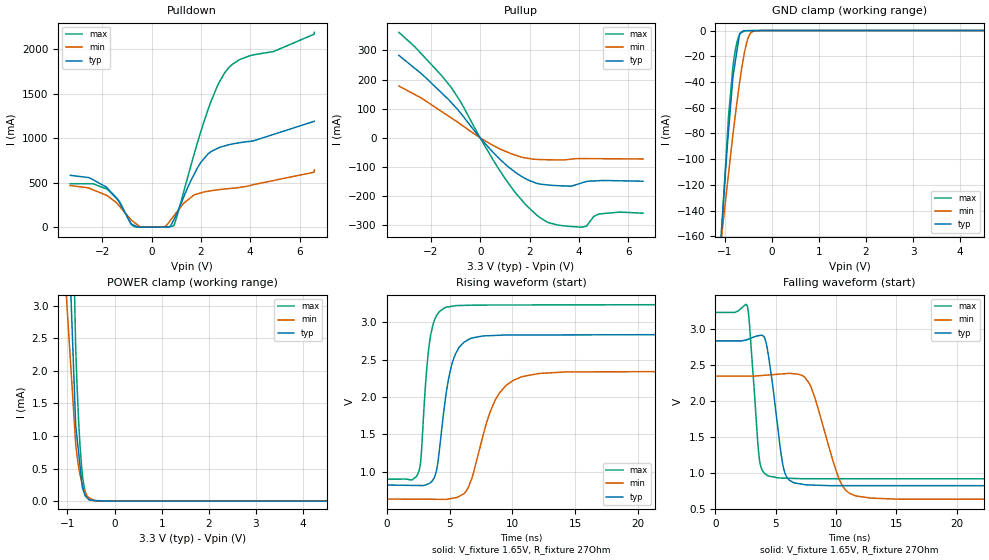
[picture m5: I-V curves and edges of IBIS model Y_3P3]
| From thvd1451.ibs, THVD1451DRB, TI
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|   Y_3P3 Model
[Model]   Y_3P3
Model_type   3-state
Polarity   Non-Inverting
Vmeas = 1.65
Vref = 1.65
Cref = 50pF
Rref = 27
|   typ   min   max
C_comp   31.02pF   29.217pF   31.597pF
|  Where Nom  PVT is Nominal Process,   3.3V,  25C
|   Fast PVT is Strong Process,   3.6V, -40C
|   Slow PVT is Weak Process,   3V, 150C
[Voltage Range]   3.3   3   3.6
|Junction Temperature
[Temperature Range]   25   150   -40
[Pullup Reference]   3.3   3   3.6
[Pulldown Reference]   -0   -0   -0
[Power Clamp Reference]   3.3   3   3.6
[GND Clamp Reference]   0   0   0
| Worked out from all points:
|   slope of the pulldown table from 0 to 0.495 V, typ, clamps not added: 418 ohm
|   slope of the pullup table from 0 to 0.495 V, typ, clamps not added: 10.5 ohm
|   GND clamp passes 1 mA (typ) near -0.63 V on its own axis
|   POWER clamp passes 1 mA (typ) near -0.80 V on its own axis
|   falling waveform, V_fixture 1.65V, R_fixture 27Ohm: 20-80 % time 911ps typ, 1.8ns min, 581ps max; typ from 2.84 V to 0.82 V
|   rising waveform, V_fixture 1.65V, R_fixture 27Ohm: 20-80 % time 1.03ns typ, 1.9ns min, 640ps max; typ from 0.822 V to 2.83 V
[Pulldown]
|   Voltage   I(typ)   I(min)   I(max)
-3.3V     582.3mA    467.5mA    487.3mA
-1.792V   436.4mA    351.7mA    425.6mA
-1.301V   273.3mA    234.6mA    288.4mA
-824.5mV  35.53mA    80.29mA    27.54mA
-542.5mV  43.41uA    19.29mA    295.2uA
506.7mV   1.255mA    3.612mA    71.17nA
885.2mV   74.4mA     120.1mA    12.22mA
2V        728.2mA    385.1mA    1.075A
2.382V    842.4mA    407.5mA    1.392A
2.954V    912.2mA    428.4mA    1.73A
3.553V    947.5mA    445.9mA    1.88A
6.6V      1.189A     644.2mA    2.189A
[GND Clamp]
|   Voltage   I(typ)   I(min)   I(max)
-3.3V     -1.548A    -990.6mA   -2.041A
-1.101V   -171.8mA   -171.2mA   -185.6mA
-1.033V   -136.5mA   -149.1mA   -136.5mA
-919.5mV  -78.47mA   -111.8mA   -67.03mA
-824.5mV  -35.9mA    -80.6mA    -27.84mA
-743.3mV  -16.65mA   -56.73mA   -9.665mA
-683.1mV  -2.377mA   -40.33mA   -3.204mA
-607.9mV  -259.9uA   -22.68mA   -874.1uA
-539.8mV  -43.77uA   -10.19mA   -189.1uA
-455.6mV  -35.02uA   -2.174mA   -132.2uA
-226.9mV  -11.24uA   -3.577uA   0A
6.6V      0A         0A         0A
[Pullup]
|   Voltage   I(typ)   I(min)   I(max)
-3.3V     282.9mA    177.7mA    361.8mA
-2.643V   237.7mA    148.1mA    311.5mA
-1.167V   120.5mA    67.89mA    171.9mA
1.011V    -89.93mA   -45.63mA   -139.8mA
1.858V    -140.8mA   -69.02mA   -230.4mA
2.379V    -157.6mA   -74.12mA   -270.8mA
3.13V     -163.8mA   -75.56mA   -298.6mA
4.126V    -154.1mA   -71.01mA   -306.1mA
4.312V    -149.6mA   -71.11mA   -302.7mA
4.606V    -147.7mA   -71.29mA   -269.5mA
4.809V    -146.8mA   -71.41mA   -261mA
6.6V      -148.6mA   -72.45mA   -258.2mA
[POWER Clamp]
|   Voltage   I(typ)   I(min)   I(max)
-3.3V     161mA      93.34mA    244.2mA
-1.071V   6.002mA    3.699mA    10.71mA
-824.7mV  1.161mA    876.2uA    2.345mA
-788.2mV  916.1uA    650.5uA    1.642mA
-763.1mV  747.1uA    528.3uA    1.236mA
-733.4mV  547.4uA    409.3uA    852.7uA
-683.9mV  214.5uA    251.3uA    413.5uA
-627.5mV  91.47uA    142.9uA    154.5uA
-541.5mV  20.13uA    53.78uA    30.12uA
-401.2mV  8.942uA    6.461uA    4.481uA
-204.7uV  0A         0A         0A
6.6V      0A         0A         0A
[Ramp]
R_load = 27
|   typ   min   max
dV/dt_r   1.2078/1.02982e-09   1.02569/1.89315e-09   1.4001/6.3862e-10
dV/dt_f   1.20985/9.08452e-10   1.03024/1.7996e-09   1.39137/5.80507e-10
[Falling Waveform]
V_fixture = 1.65V
V_fixture_min = 1.5V
V_fixture_max = 1.8V
R_fixture = 27Ohm
C_fixture = 0F
|   Time   V(typ)   V(min)   V(max)
0s        2.836V     2.347V     3.234V
2.647ns   2.855V     2.346V     3.326V
3.637ns   2.911V     2.352V     1.212V
4.319ns   2.719V     2.361V     962.4mV
5.587ns   1.119V     2.377V     925.5mV
6.442ns   866.2mV    2.38V      920.8mV
7.843ns   829.5mV    2.226V     916.8mV
10.06ns   819.8mV    1.003V     916.6mV
11.12ns   819.8mV    713.7mV    916.5mV
30ns      820mV      629.6mV    914.9mV
[Rising Waveform]
V_fixture = 1.65V
V_fixture_min = 1.5V
V_fixture_max = 1.8V
R_fixture = 27Ohm
C_fixture = 0F
|   Time   V(typ)   V(min)   V(max)
0s        822.3mV    634.2mV    901.7mV
2.542ns   816.2mV    632.6mV    995.4mV
3.456ns   850.3mV    632mV      2.781V
3.966ns   1.018V     631.7mV    3.086V
4.614ns   1.9V       631.2mV    3.191V
5.222ns   2.457V     644.6mV    3.213V
6.145ns   2.731V     707mV      3.223V
8.588ns   2.822V     1.94V      3.228V
10.68ns   2.827V     2.265V     3.229V
30ns      2.835V     2.344V     3.235V
